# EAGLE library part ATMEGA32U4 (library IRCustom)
http://www.ladyada.net/library/eagle
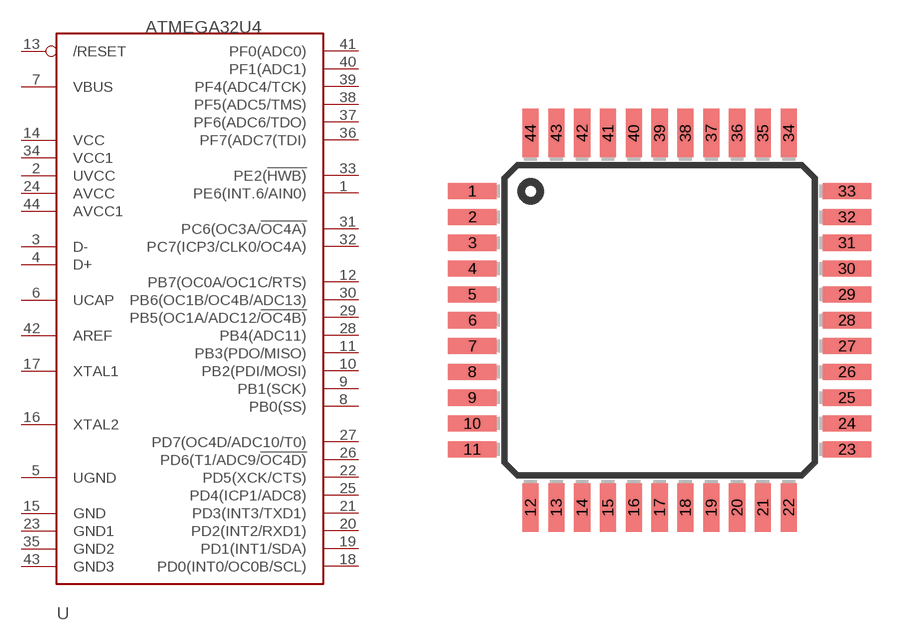
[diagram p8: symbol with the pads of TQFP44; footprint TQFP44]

Designator prefix -

## ATMEGA32U4-AU  [TQFP44]
1  PE6(INT.6/AIN0)
2  UVCC
3  D-
4  D+
5  UGND
6  UCAP
7  VBUS
8  PB0(SS)
9  PB1(SCK)
10  PB2(PDI/MOSI)
11  PB3(PDO/MISO)
12  PB7(OC0A/OC1C/RTS)
13  /RESET
14  VCC
15  GND
16  XTAL2
17  XTAL1
18  PD0(INT0/OC0B/SCL)
19  PD1(INT1/SDA)
20  PD2(INT2/RXD1)
21  PD3(INT3/TXD1)
22  PD5(XCK/CTS)
23  GND1
24  AVCC
25  PD4(ICP1/ADC8)
26  PD6(T1/ADC9/!OC4D)
27  PD7(OC4D/ADC10/T0)
28  PB4(ADC11)
29  PB5(OC1A/ADC12/!OC4B)
30  PB6(OC1B/OC4B/ADC13)
31  PC6(OC3A/!OC4A)
32  PC7(ICP3/CLK0/OC4A)
33  PE2(!HWB)
34  VCC1
35  GND2
36  PF7(ADC7(TDI)
37  PF6(ADC6/TDO)
38  PF5(ADC5/TMS)
39  PF4(ADC4/TCK)
40  PF1(ADC1)
41  PF0(ADC0)
42  AREF
43  GND3
44  AVCC1

## Footprint TQFP44 (pad centres in mm)
smd 1.5 x 0.5: 1 -5.8,4; 2 -5.8,3.2; 3 -5.8,2.4; 4 -5.8,1.6; 5 -5.8,0.8; 6 -5.8,0; 7 -5.8,-0.8; 8 -5.8,-1.6; 9 -5.8,-2.4; 10 -5.8,-3.2; 11 -5.8,-4; 23 5.8,-4; 24 5.8,-3.2; 25 5.8,-2.4; 26 5.8,-1.6; 27 5.8,-0.8; 28 5.8,0; 29 5.8,0.8; 30 5.8,1.6; 31 5.8,2.4; 32 5.8,3.2; 33 5.8,4
smd 0.5 x 1.5: 12 -4,-5.8; 13 -3.2,-5.8; 14 -2.4,-5.8; 15 -1.6,-5.8; 16 -0.8,-5.8; 17 0,-5.8; 18 0.8,-5.8; 19 1.6,-5.8; 20 2.4,-5.8; 21 3.2,-5.8; 22 4,-5.8; 34 4,5.8; 35 3.2,5.8; 36 2.4,5.8; 37 1.6,5.8; 38 0.8,5.8; 39 0,5.8; 40 -0.8,5.8; 41 -1.6,5.8; 42 -2.4,5.8; 43 -3.2,5.8; 44 -4,5.8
